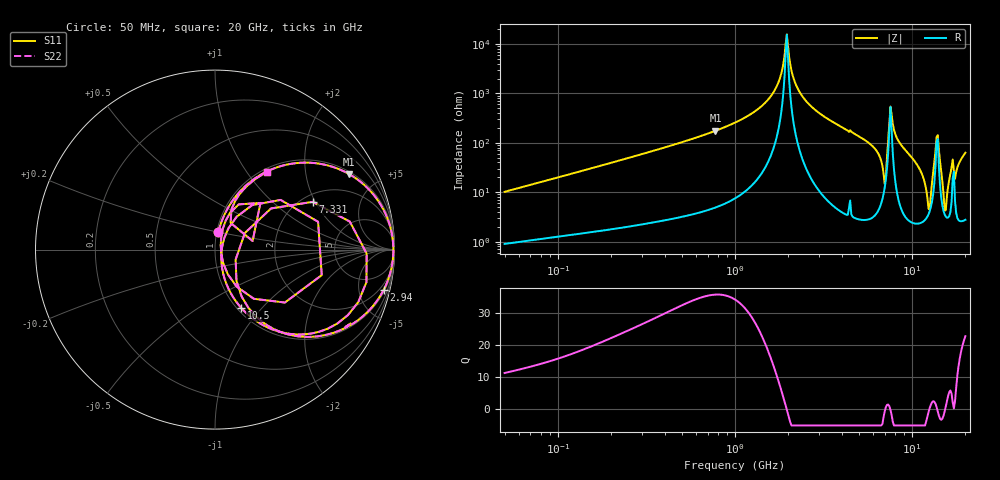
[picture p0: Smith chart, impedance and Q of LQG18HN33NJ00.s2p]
!Murata Part Number: LQG18HN33NJ00
!These Parameters are Measured in Series Mode Connection
!  o--[Z]--o
!Port1  Port2
!  o-------o
!Freq. Start=50[MHz] Stop=20[GHz], 401[Steps]
# Hz S RI R 50
!Freq.(Hz) S11(Real) S11(Imag) S21(Real) S21(Imag) S12(Real) S12(Imag) S22(Real) S22(Imag)
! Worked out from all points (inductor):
!   401 points, 50 MHz to 20 GHz, reference 50 ohm
!   read as one part in series: L = 32 nH near 51.52 MHz
!   highest Q = 35.7 at 775.2 MHz (marker M1), where L = 35.9 nH
!   self-resonance near 1.933 GHz
!   S11 on the Smith chart (normalised r, x): 50 MHz: 1.02, +0.20; 2.94 GHz: 1.23, -8.36; 7.331 GHz: 2.27, +1.91; 10.5 GHz: 1.05, -0.78; 20 GHz: 1.06, +1.26
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5e7  0.0188 0.0987  0.9812 -0.0987  0.9812 -0.0987  0.0188 0.0987
1.364002e8  0.0793 0.2444  0.9207 -0.2444  0.9207 -0.2444  0.0793 0.2444
3.721004e8  0.3606 0.4632  0.6394 -0.4632  0.6394 -0.4632  0.3606 0.4632
7.751977e8  0.7475 0.4207  0.2525 -0.4207  0.2525 -0.4207  0.7475 0.4207
1e9  0.8604 0.3322  0.1396 -0.3322  0.1396 -0.3322  0.8604 0.3322
1.614971e9  0.982 0.1038  0.018 -0.1038  0.018 -0.1038  0.982 0.1038
1.962148e9  0.9936 -0.00061  0.00635 0.00061  0.00635 0.00061  0.9936 -0.00061
2.211938e9  0.9894 -0.0663  0.0106 0.0663  0.0106 0.0663  0.9894 -0.0663
2.728004e9  0.9591 -0.1822  0.0409 0.1822  0.0409 0.1822  0.9591 -0.1822
2.940159e9  0.9404 -0.2234  0.0596 0.2234  0.0596 0.2234  0.9404 -0.2234
6.034176e9  0.4101 -0.4732  0.5899 0.4732  0.5899 0.4732  0.4101 -0.4732
6.905011e9  0.1195 -0.1742  0.8805 0.1742  0.8805 0.1742  0.1195 -0.1742
7.331367e9  0.5436 0.266  0.4564 -0.266  0.4564 -0.266  0.5436 0.266
7.442007e9  0.7512 0.156  0.2488 -0.156  0.2488 -0.156  0.7512 0.156
8.264682e9  0.5795 -0.458  0.4205 0.458  0.4205 0.458  0.5795 -0.458
1.050288e10  0.1475 -0.3263  0.8525 0.3263  0.8525 0.3263  0.1475 -0.3263
1.238412e10  0.0353 -0.0278  0.9647 0.0278  0.9647 0.0278  0.0353 -0.0278
1.334722e10  0.2075 0.248  0.7925 -0.248  0.7925 -0.248  0.2075 0.248
1.396067e10  0.5947 -0.1423  0.4053 0.1423  0.4053 0.1423  0.5947 -0.1423
1.550395e10  0.0318 0.0282  0.9682 -0.0282  0.9682 -0.0282  0.0318 0.0282
1.646126e10  0.0848 0.206  0.9152 -0.206  0.9152 -0.206  0.0848 0.206
2e10  0.2925 0.4335  0.7075 -0.4335  0.7075 -0.4335  0.2925 0.4335
